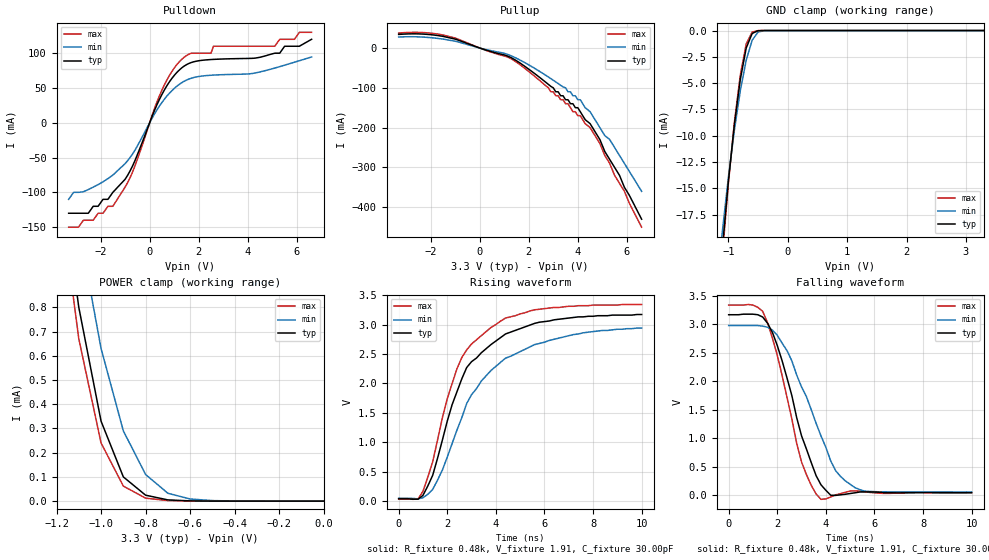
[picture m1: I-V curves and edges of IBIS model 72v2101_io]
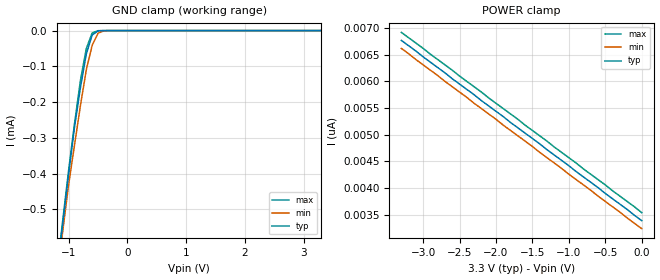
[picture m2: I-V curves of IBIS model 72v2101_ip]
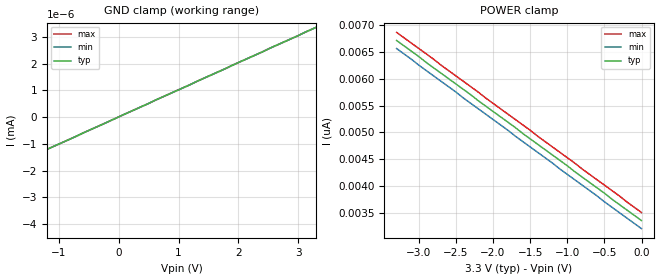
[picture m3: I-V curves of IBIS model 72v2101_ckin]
| IBIS file 72v2111.ibs created by s2ibis2 version 1.1
| North Carolina State University Electronics Research Laboratory  1995
[IBIS ver]   2.1
[File name]   72v2111.ibs
[File Rev]   1.1
[Date]   03/16/00
[Source]   Integrated Device Technology, Inc.
[Notes]   1.Temperatures: typ=25C, min=100C, max=0C 2.Cemos8 5vv
   process. 3.RRmp rates based on 50 ohm load.
[Disclaimer] Integrated Device Technology, Inc. ("IDT") hereby grants the
   user of this IBIS model a non-exclusive, nontransferable
   license to use this IBIS model under the following terms. The
   user is granted this license only to use the IBIS model and is
   not granted rights to sell, copy (except as needed to run the
   IBIS model), rent, lease or sub-license the IBIS model in
   whole or in part, or in modified form to anyone. The User may
   modify the IBIS model to suit its specific applications, but
   rights to derivative works and such modifications shall belong
   to IDT. This IBIS model is provided on an AS IS" basis and IDT
   makes absolutely no warranty with respect to the information
   contained herein. IDT DISCLAIMS AND CUSTOMER WAIVES ALL
   WARRANTIES, EXPRESS AND IMPLIED, INCLUDING WARRANTIES OF
   MERCHANTABILITY AND FITNESS FOR A PARTICULAR PURPOSE. THE
   ENTIRE RISK AS TO QUALITY AND PERFORMANCE IS WITH THE USER
   ACCORDINGLY, IN NO EVENT SHALL IDT BE LIABLE FOR ANY DIRECT OR
   INDIRECT DAMAGES, WHETHER IN CONTRACT OR TORT, INCLUDING ANY
   LOST PROFITS OR OTHER INCIDENTAL, CONSEQUENTIAL, EXEMPLARY, OR
   PUNITIVE DAMAGES ARISING OUT OF THE USE OR APPLICATION OF THE
   IBIS model. Further, IDT reserves the right to make changes
   without notice to any product herein to improve reliability,
   function, or design. IDT does not convey any license under
   patent rights or any other intellectual property rights,
   including those of third parties. IDT is not obligated to
   provide maintenance or support for the licensed IBIS model.
[Copyright]   Copyright 2000, Integrated Device Technology, Inc. all rights
   reserved
|   Component idt72v2111pn64
[Component]   idt72v2111pn64
[Manufacturer]   Integrated Device Technology
[Package]
| variable   typ   min   max
R_pkg   100.00m   50.00m   0.30
L_pkg   4.50nH   4.20nH   4.80nH
C_pkg   0.40pF   50.00fF   0.90pF
[Pin]  signal_name   model_name   R_pin   L_pin   C_pin
1   WEN   72v2101_ip
2   SEN   72v2101_ip
3   GND   GND
4   VDD   POWER
5   VDD   POWER
6   GND   GND
7   GND   GND
8   GND   GND
9   GND   GND
10   GND   GND
11   GND   GND
12   GND   GND
13   GND   GND
14   GND   GND
15   D8   72v2101_ip
16   D7   72v2101_ip
17   D6   72v2101_ip
18   D5   72v2101_ip
19   D4   72v2101_ip
20   D3   72v2101_ip
21   D2   72v2101_ip
22   D1   72v2101_ip
23   D0   72v2101_ip
24   GND   GND
25   Q0   72v2101_io
26   Q1   72v2101_io
27   GND   GND
28   Q2   72v2101_io
29   Q3   72v2101_io
30   VDD   POWER
31   Q4   72v2101_io
32   Q5   72v2101_io
33   GND   GND
34   Q6   72v2101_io
35   Q7   72v2101_io
36   Q8   72v2101_io
37   NC   NC
38   NC   NC
39   GND   GND
40   NC   NC
41   NC   NC
42   NC   NC
43   VDD   POWER
44   NC   NC
45   NC   NC
46   GND   GND
47   NC   NC
48   NC   NC
49   OE   72v2101_ckin
50   RT   72v2101_ip
51   REN   72v2101_ip
52   RCLK   72v2101_ckin
53   EF_OR   72v2101_io
54   PAE   72v2101_io
55   VDD   POWER
56   HF   72v2101_io
57   PAF   72v2101_io
58   FF_IR   72v2101_io
59   GND   GND
60   FWFT_SI   72v2101_ip
61   LD   72v2101_ip
62   MRS   72v2101_ip
63   PRS   72v2101_ip
64   WCLK   72v2101_ckin
| Models and submodels in the file (3): 72v2101_io (I/O), 72v2101_ip (Input), 72v2101_ckin (Input)
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| dout dout   dummy_model
| oen  oen   dummy_model
|   Model 72v2101_io
[Model]   72v2101_io
Model_type   I/O
Polarity   Inverting
Enable   Active-Low
Vinl =  0.000V
Vinh =   3.30V
Vmeas =   1.50V
C_comp   3.00pF   NA   NA
[Temperature Range]   25.00   100.00   0.000
[Voltage Range]   3.30V   3.15V   3.45V
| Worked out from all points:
|   slope of the pulldown table from 0 to 0.495 V, typ, clamps not added: 12.3 ohm
|   slope of the pullup table from 0 to 0.495 V, typ, clamps not added: 51.3 ohm
|   GND clamp passes 1 mA (typ) near -0.65 V on its own axis
|   POWER clamp passes 1 mA (typ) near -1.13 V on its own axis
|   rising waveform, R_fixture 0.48k, V_fixture 1.91, C_fixture 30.00pF: 20-80 % time 1.91ns typ, 2.32ns min, 1.61ns max; typ from 0.041 V to 3.17 V
|   falling waveform, R_fixture 0.48k, V_fixture 1.91, C_fixture 30.00pF: 20-80 % time 1.26ns typ, 1.61ns min, 1.07ns max; typ from 3.17 V to 0.041 V
[Pulldown]
| voltage   I(typ)   I(min)   I(max)
-3.3V     -130mA     -110mA     -150mA
-2.5V     -130mA     -96mA      -140mA
-1.5V     -100mA     -75.17mA   -120mA
-700mV    -62.36mA   -44.99mA   -71.09mA
600mV     47.15mA    33.89mA    54.42mA
1.4V      81.31mA    59.52mA    94.07mA
2.5V      90.89mA    68.31mA    100mA
2.6V      91.1mA     68.53mA    110mA
5.1V      100mA      78.64mA    110mA
5.3V      100mA      80.67mA    120mA
5.5V      110mA      82.76mA    120mA
6.6V      120mA      94.56mA    130mA
[Pullup]
| voltage   I(typ)   I(min)   I(max)
-3.3V     34.07mA    27.51mA    37.51mA
-2.1V     33.99mA    26.45mA    37.82mA
-1V       22.31mA    16.98mA    25mA
1.2V      -21.92mA   -17.57mA   -24.6mA
1.9V      -48.75mA   -38.92mA   -54.09mA
3.5V      -130mA     -100mA     -140mA
4V        -150mA     -130mA     -170mA
4.5V      -190mA     -160mA     -200mA
4.9V      -230mA     -200mA     -240mA
5.3V      -280mA     -230mA     -290mA
5.7V      -320mA     -270mA     -340mA
6.6V      -430mA     -360mA     -450mA
[GND_clamp]
| voltage   I(typ)   I(min)   I(max)
-3.3V     -250mA     -200mA     -270mA
-1.1V     -20.55mA   -18.99mA   -21.24mA
-1V       -14.32mA   -13.94mA   -14.5mA
-900mV    -8.97mA    -9.49mA    -8.76mA
-800mV    -4.66mA    -5.74mA    -4.24mA
-700mV    -1.66mA    -2.81mA    -1.27mA
-600mV    -280uA     -920uA     -150uA
-500mV    -18.22uA   -150uA     -6.63uA
-400mV    -540nA     -12.94uA   -120nA
3.3V      3.52nA     10.49nA    3.51nA
[POWER_clamp]
| voltage   I(typ)   I(min)   I(max)
-3.3V     26.68mA    22.13mA    28.89mA
-1.2V     1.48mA     1.76mA     1.37mA
-1.1V     800uA      1.13mA     670uA
-1V       330uA      630uA      240uA
-900mV    100uA      290uA      62.08uA
-800mV    24.53uA    110uA      12.31uA
-700mV    5.11uA     32.54uA    2.24uA
-600mV    1uA        8.76uA     380nA
-400mV    28.8nA     520nA      10.2nA
0V        3.52nA     3.39nA     3.68nA
[Ramp]
| variable   typ   min   max
dV/dt_r   1.04/0.53n   0.91/0.75n   1.14/0.48n
dV/dt_f   1.57/0.96n   1.36/1.39n   1.69/0.75n
R_load = 50.00
[Rising Waveform]
R_fixture = 0.48k
V_fixture = 1.91
V_fixture_min = 1.72
V_fixture_max = 2.10
C_fixture = 30.00pF
R_dut = 100.00m
L_dut = 4.00nH
C_dut = 0.60pF
| time   V(typ)   V(min)   V(max)
0s        41.49mV    52.25mV    39.66mV
800ps     35.72mV    41.52mV    41.7mV
1.4ns     440mV      200mV      670mV
2ns       1.36V      750mV      1.74V
2.4ns     1.86V      1.21V      2.25V
2.8ns     2.27V      1.66V      2.57V
3.8ns     2.66V      2.22V      2.95V
4.4ns     2.84V      2.43V      3.11V
6.2ns     3.06V      2.73V      3.28V
10ns      3.17V      2.94V      3.34V
[Falling Waveform]
R_fixture = 0.48k
V_fixture = 1.91
V_fixture_min = 1.72
V_fixture_max = 2.10
C_fixture = 30.00pF
R_dut = 100.00m
L_dut = 4.00nH
C_dut = 0.60pF
| time   V(typ)   V(min)   V(max)
0s        3.17V      2.98V      3.34V
1.4ns     3.13V      2.97V      3.23V
2ns       2.63V      2.81V      2.46V
2.6ns     1.75V      2.36V      1.34V
3ns       1.04V      1.9V       580mV
3.4ns     570mV      1.5V       170mV
3.8ns     180mV      1.04V      -75.52mV
4.4ns     -6.44mV    430mV      1.79mV
5.4ns     53.55mV    94.27mV    69.91mV
10ns      41.47mV    52.47mV    40.14mV
|   Model 72v2101_ip
[Model]   72v2101_ip
Model_type   Input
Vinl =   0.80V
Vinh =   2.20V
Vmeas =   1.50V
C_comp   3.00pF   NA   NA
[Temperature Range]   25.00   100.00   0.000
[Voltage Range]   3.30V   3.15V   3.45V
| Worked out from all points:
|   GND clamp passes 1 mA (typ) near -1.41 V on its own axis
[GND_clamp]
| voltage   I(typ)   I(min)   I(max)
-3.3V     -4.63mA    -4.57mA    -4.66mA
-1.2V     -680uA     -690uA     -670uA
-1.1V     -540uA     -560uA     -530uA
-1V       -400uA     -430uA     -390uA
-900mV    -270uA     -320uA     -260uA
-800mV    -160uA     -210uA     -140uA
-700mV    -65.76uA   -110uA     -50.5uA
-600mV    -12.68uA   -41.3uA    -6.8uA
-500mV    -820nA     -7.39uA    -280nA
-400mV    -21.8nA    -610nA     -4.72nA
3.3V      3.39nA     3.39nA     3.39nA
[POWER_clamp]
| voltage   I(typ)   I(min)   I(max)
-3.3V     6.77nA     6.62nA     6.92nA
-2.1V     5.54nA     5.39nA     5.69nA
-1.7V     5.13nA     4.98nA     5.29nA
0V        3.39nA     3.24nA     3.54nA
|   Model 72v2101_ckin
[Model]   72v2101_ckin
Model_type   Input
Vinl =   0.80V
Vinh =   2.20V
Vmeas =   1.50V
C_comp   3.00pF   NA   NA
[Temperature Range]   25.00   100.00   0.000
[Voltage Range]   3.30V   3.15V   3.45V
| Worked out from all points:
|   GND clamp passes 1 mA (typ) near -2.33 V on its own axis
[GND_clamp]
| voltage   I(typ)   I(min)   I(max)
-3.3V     -3.42mA    -3.29mA    -3.46mA
-1.6V     -41.43nA   -1.14uA    -9.79nA
-1.5V     -2.1nA     -48.95nA   -1.59nA
-1.4V     -1.42nA    -2.83nA    -1.42nA
-1.3V     -1.31nA    -1.36nA    -1.31nA
-1.2V     -1.21nA    -1.21nA    -1.21nA
3.3V      3.36nA     3.36nA     3.36nA
[POWER_clamp]
| voltage   I(typ)   I(min)   I(max)
-3.3V     6.71nA     6.56nA     6.86nA
-600mV    3.97nA     3.82nA     4.12nA
-500mV    3.87nA     3.71nA     4.02nA
0V        3.36nA     3.21nA     3.51nA
